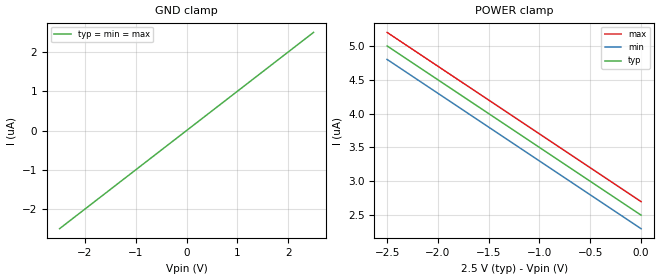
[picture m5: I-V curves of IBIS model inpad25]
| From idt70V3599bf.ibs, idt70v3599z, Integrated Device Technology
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|   Model inpad25
[Model]   inpad25
Model_type   Input
Vinl =  0.70000V
Vinh =  1.70000V
C_comp   4.50000pF   NA   NA
[Temperature Range]   25.00000   100.00000   0.000
[Voltage Range]   2.50000V   2.30000V   2.70000V
[GND_clamp]
| voltage   I(typ)   I(min)   I(max)
-2.5V     -2.5uA     -2.5uA     -2.5uA
1.9V      1.9uA      1.9uA      1.9uA
2.4V      2.4uA      2.4uA      2.4uA
2.5V      2.5uA      2.5uA      2.5uA
[POWER_clamp]
| voltage   I(typ)   I(min)   I(max)
-2.5V     5uA        4.8uA      5.2uA
-2.4V     4.9uA      4.7uA      5.1uA
-2.1V     4.6uA      4.4uA      4.8uA
0V        2.5uA      2.3uA      2.7uA
